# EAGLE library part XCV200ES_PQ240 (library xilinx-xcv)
xcv200es_pq240 edit this description Auto generated by make-symbol-device-package-bsdl.ulp Rev. 26 Source: xcv200es_pq240.bsd
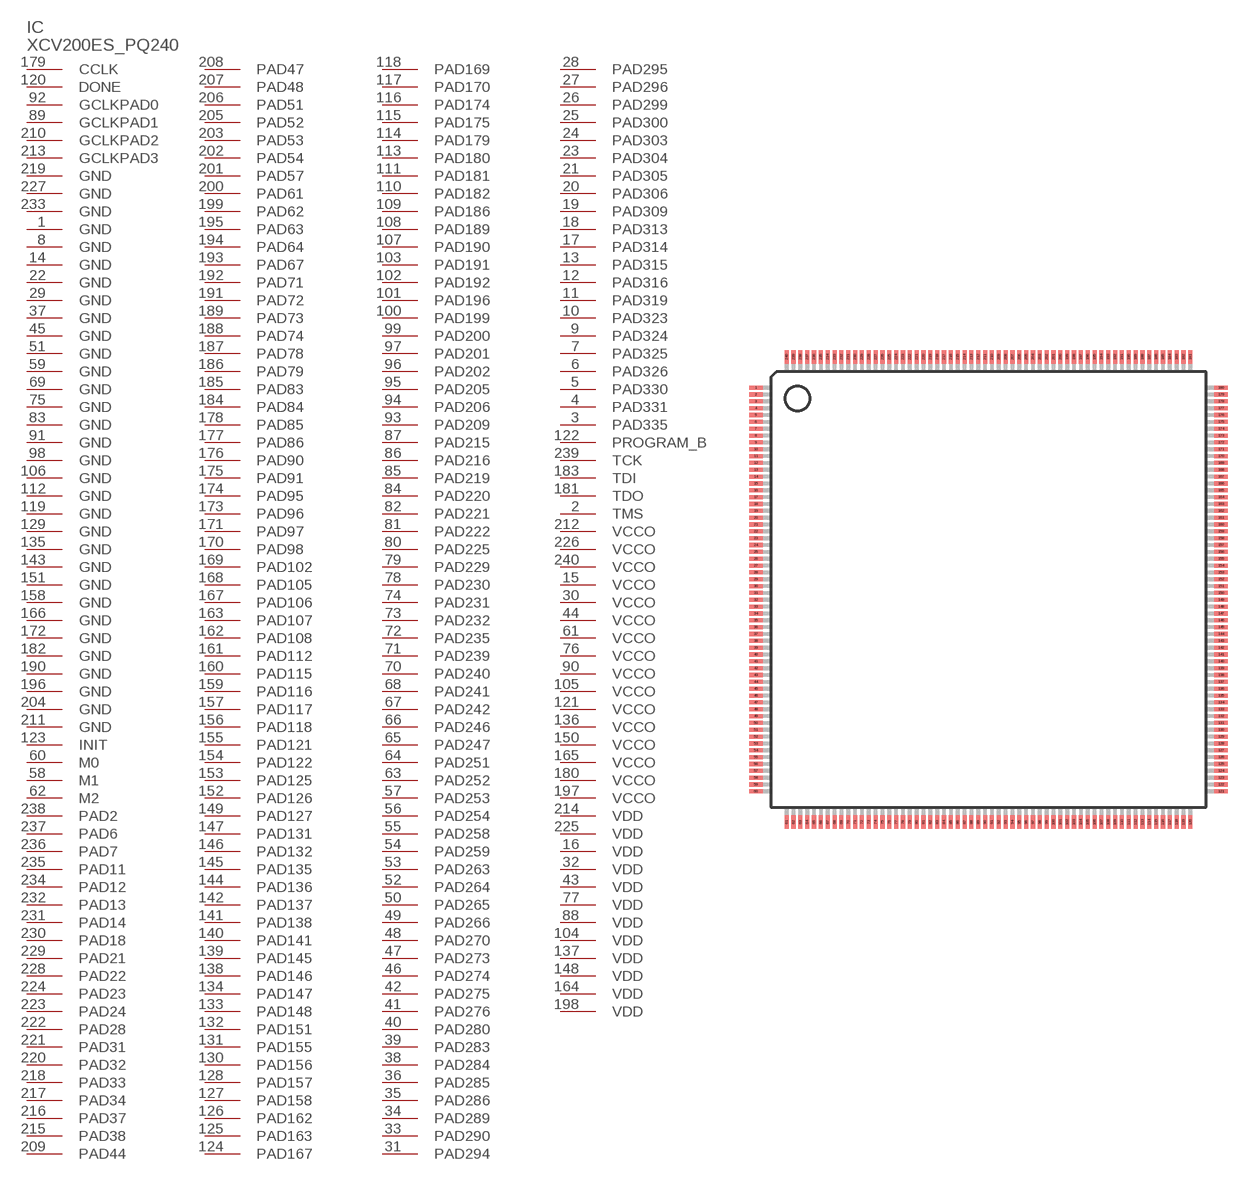
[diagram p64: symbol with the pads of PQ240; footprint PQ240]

Designator prefix IC

## XCV200ES_PQ240 (OC_FARNELL: unknown; OC_NEWARK: unknown)  [PQ240]
1  GND  pwr
2  TMS  in
3  PAD335
4  PAD331
5  PAD330
6  PAD326
7  PAD325
8  GND  pwr
9  PAD324
10  PAD323
11  PAD319
12  PAD316
13  PAD315
14  GND  pwr
15  VCCO  pwr
16  VDD  pwr
17  PAD314
18  PAD313
19  PAD309
20  PAD306
21  PAD305
22  GND  pwr
23  PAD304
24  PAD303
25  PAD300
26  PAD299
27  PAD296
28  PAD295
29  GND  pwr
30  VCCO  pwr
31  PAD294
32  VDD  pwr
33  PAD290
34  PAD289
35  PAD286
36  PAD285
37  GND  pwr
38  PAD284
39  PAD283
40  PAD280
41  PAD276
42  PAD275
43  VDD  pwr
44  VCCO  pwr
45  GND  pwr
46  PAD274
47  PAD273
48  PAD270
49  PAD266
50  PAD265
51  GND  pwr
52  PAD264
53  PAD263
54  PAD259
55  PAD258
56  PAD254
57  PAD253
58  M1  in
59  GND  pwr
60  M0  in
61  VCCO  pwr
62  M2  in
63  PAD252
64  PAD251
65  PAD247
66  PAD246
67  PAD242
68  PAD241
69  GND  pwr
70  PAD240
71  PAD239
72  PAD235
73  PAD232
74  PAD231
75  GND  pwr
76  VCCO  pwr
77  VDD  pwr
78  PAD230
79  PAD229
80  PAD225
81  PAD222
82  PAD221
83  GND  pwr
84  PAD220
85  PAD219
86  PAD216
87  PAD215
88  VDD  pwr
89  GCLKPAD1  in
90  VCCO  pwr
91  GND  pwr
92  GCLKPAD0  in
93  PAD209
94  PAD206
95  PAD205
96  PAD202
97  PAD201
98  GND  pwr
99  PAD200
100  PAD199
101  PAD196
102  PAD192
103  PAD191
104  VDD  pwr
105  VCCO  pwr
106  GND  pwr
107  PAD190
108  PAD189
109  PAD186
110  PAD182
111  PAD181
112  GND  pwr
113  PAD180
114  PAD179
115  PAD175
116  PAD174
117  PAD170
118  PAD169
119  GND  pwr
120  DONE
121  VCCO  pwr
122  PROGRAM_B  in
123  INIT
124  PAD167
125  PAD163
126  PAD162
127  PAD158
128  PAD157
129  GND  pwr
130  PAD156
131  PAD155
132  PAD151
133  PAD148
134  PAD147
135  GND  pwr
136  VCCO  pwr
137  VDD  pwr
138  PAD146
139  PAD145
140  PAD141
141  PAD138
142  PAD137
143  GND  pwr
144  PAD136
145  PAD135
146  PAD132
147  PAD131
148  VDD  pwr
149  PAD127
150  VCCO  pwr
151  GND  pwr
152  PAD126
153  PAD125
154  PAD122
155  PAD121
156  PAD118
157  PAD117
158  GND  pwr
159  PAD116
160  PAD115
161  PAD112
162  PAD108
163  PAD107
164  VDD  pwr
165  VCCO  pwr
166  GND  pwr
167  PAD106
168  PAD105
169  PAD102
170  PAD98
171  PAD97
172  GND  pwr
173  PAD96
174  PAD95
175  PAD91
176  PAD90
177  PAD86
178  PAD85
179  CCLK
180  VCCO  pwr
181  TDO  out
182  GND  pwr
183  TDI  in
184  PAD84
185  PAD83
186  PAD79
187  PAD78
188  PAD74
189  PAD73
190  GND  pwr
191  PAD72
192  PAD71
193  PAD67
194  PAD64
195  PAD63
196  GND  pwr
197  VCCO  pwr
198  VDD  pwr
199  PAD62
200  PAD61
201  PAD57
202  PAD54
203  PAD53
204  GND  pwr
205  PAD52
206  PAD51
207  PAD48
208  PAD47
209  PAD44
210  GCLKPAD2  in
211  GND  pwr
212  VCCO  pwr
213  GCLKPAD3  in
214  VDD  pwr
215  PAD38
216  PAD37
217  PAD34
218  PAD33
219  GND  pwr
220  PAD32
221  PAD31
222  PAD28
223  PAD24
224  PAD23
225  VDD  pwr
226  VCCO  pwr
227  GND  pwr
228  PAD22
229  PAD21
230  PAD18
231  PAD14
232  PAD13
233  GND  pwr
234  PAD12
235  PAD11
236  PAD7
237  PAD6
238  PAD2
239  TCK  in
240  VCCO  pwr

## Footprint PQ240 (pad centres in mm)
PQ240 Auto generated by make-symbol-device-package-bsdl.ulp Rev. 26
smd 1 x 0.3: 1 -17,14.75; 2 -17,14.25; 3 -17,13.75; 4 -17,13.25; 5 -17,12.75; 6 -17,12.25; 7 -17,11.75; 8 -17,11.25; 9 -17,10.75; 10 -17,10.25; 11 -17,9.75; 12 -17,9.25; 13 -17,8.75; 14 -17,8.25; 15 -17,7.75; 16 -17,7.25; 17 -17,6.75; 18 -17,6.25; 19 -17,5.75; 20 -17,5.25; 21 -17,4.75; 22 -17,4.25; 23 -17,3.75; 24 -17,3.25; 25 -17,2.75; 26 -17,2.25; 27 -17,1.75; 28 -17,1.25; 29 -17,0.75; 30 -17,0.25; 31 -17,-0.25; 32 -17,-0.75; 33 -17,-1.25; 34 -17,-1.75; 35 -17,-2.25; 36 -17,-2.75; 37 -17,-3.25; 38 -17,-3.75; 39 -17,-4.25; 40 -17,-4.75; 41 -17,-5.25; 42 -17,-5.75; 43 -17,-6.25; 44 -17,-6.75; 45 -17,-7.25; 46 -17,-7.75; 47 -17,-8.25; 48 -17,-8.75; 49 -17,-9.25; 50 -17,-9.75; 51 -17,-10.25; 52 -17,-10.75; 53 -17,-11.25; 54 -17,-11.75; 55 -17,-12.25; 56 -17,-12.75; 57 -17,-13.25; 58 -17,-13.75; 59 -17,-14.25; 60 -17,-14.75; 121 17,-14.75; 122 17,-14.25; 123 17,-13.75; 124 17,-13.25; 125 17,-12.75; 126 17,-12.25; 127 17,-11.75; 128 17,-11.25; 129 17,-10.75; 130 17,-10.25; 131 17,-9.75; 132 17,-9.25; 133 17,-8.75; 134 17,-8.25; 135 17,-7.75; 136 17,-7.25; 137 17,-6.75; 138 17,-6.25; 139 17,-5.75; 140 17,-5.25; 141 17,-4.75; 142 17,-4.25; 143 17,-3.75; 144 17,-3.25; 145 17,-2.75; 146 17,-2.25; 147 17,-1.75; 148 17,-1.25; 149 17,-0.75; 150 17,-0.25; 151 17,0.25; 152 17,0.75; 153 17,1.25; 154 17,1.75; 155 17,2.25; 156 17,2.75; 157 17,3.25; 158 17,3.75; 159 17,4.25; 160 17,4.75; 161 17,5.25; 162 17,5.75; 163 17,6.25; 164 17,6.75; 165 17,7.25; 166 17,7.75; 167 17,8.25; 168 17,8.75; 169 17,9.25; 170 17,9.75; 171 17,10.25; 172 17,10.75; 173 17,11.25; 174 17,11.75; 175 17,12.25; 176 17,12.75; 177 17,13.25; 178 17,13.75; 179 17,14.25; 180 17,14.75
smd 0.3 x 1: 61 -14.75,-17; 62 -14.25,-17; 63 -13.75,-17; 64 -13.25,-17; 65 -12.75,-17; 66 -12.25,-17; 67 -11.75,-17; 68 -11.25,-17; 69 -10.75,-17; 70 -10.25,-17; 71 -9.75,-17; 72 -9.25,-17; 73 -8.75,-17; 74 -8.25,-17; 75 -7.75,-17; 76 -7.25,-17; 77 -6.75,-17; 78 -6.25,-17; 79 -5.75,-17; 80 -5.25,-17; 81 -4.75,-17; 82 -4.25,-17; 83 -3.75,-17; 84 -3.25,-17; 85 -2.75,-17; 86 -2.25,-17; 87 -1.75,-17; 88 -1.25,-17; 89 -0.75,-17; 90 -0.25,-17; 91 0.25,-17; 92 0.75,-17; 93 1.25,-17; 94 1.75,-17; 95 2.25,-17; 96 2.75,-17; 97 3.25,-17; 98 3.75,-17; 99 4.25,-17; 100 4.75,-17; 101 5.25,-17; 102 5.75,-17; 103 6.25,-17; 104 6.75,-17; 105 7.25,-17; 106 7.75,-17; 107 8.25,-17; 108 8.75,-17; 109 9.25,-17; 110 9.75,-17; 111 10.25,-17; 112 10.75,-17; 113 11.25,-17; 114 11.75,-17; 115 12.25,-17; 116 12.75,-17; 117 13.25,-17; 118 13.75,-17; 119 14.25,-17; 120 14.75,-17; 181 14.75,17; 182 14.25,17; 183 13.75,17; 184 13.25,17; 185 12.75,17; 186 12.25,17; 187 11.75,17; 188 11.25,17; 189 10.75,17; 190 10.25,17; 191 9.75,17; 192 9.25,17; 193 8.75,17; 194 8.25,17; 195 7.75,17; 196 7.25,17; 197 6.75,17; 198 6.25,17; 199 5.75,17; 200 5.25,17; 201 4.75,17; 202 4.25,17; 203 3.75,17; 204 3.25,17; 205 2.75,17; 206 2.25,17; 207 1.75,17; 208 1.25,17; 209 0.75,17; 210 0.25,17; 211 -0.25,17; 212 -0.75,17; 213 -1.25,17; 214 -1.75,17; 215 -2.25,17; 216 -2.75,17; 217 -3.25,17; 218 -3.75,17; 219 -4.25,17; 220 -4.75,17; 221 -5.25,17; 222 -5.75,17; 223 -6.25,17; 224 -6.75,17; 225 -7.25,17; 226 -7.75,17; 227 -8.25,17; 228 -8.75,17; 229 -9.25,17; 230 -9.75,17; 231 -10.25,17; 232 -10.75,17; 233 -11.25,17; 234 -11.75,17; 235 -12.25,17; 236 -12.75,17; 237 -13.25,17; 238 -13.75,17; 239 -14.25,17; 240 -14.75,17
